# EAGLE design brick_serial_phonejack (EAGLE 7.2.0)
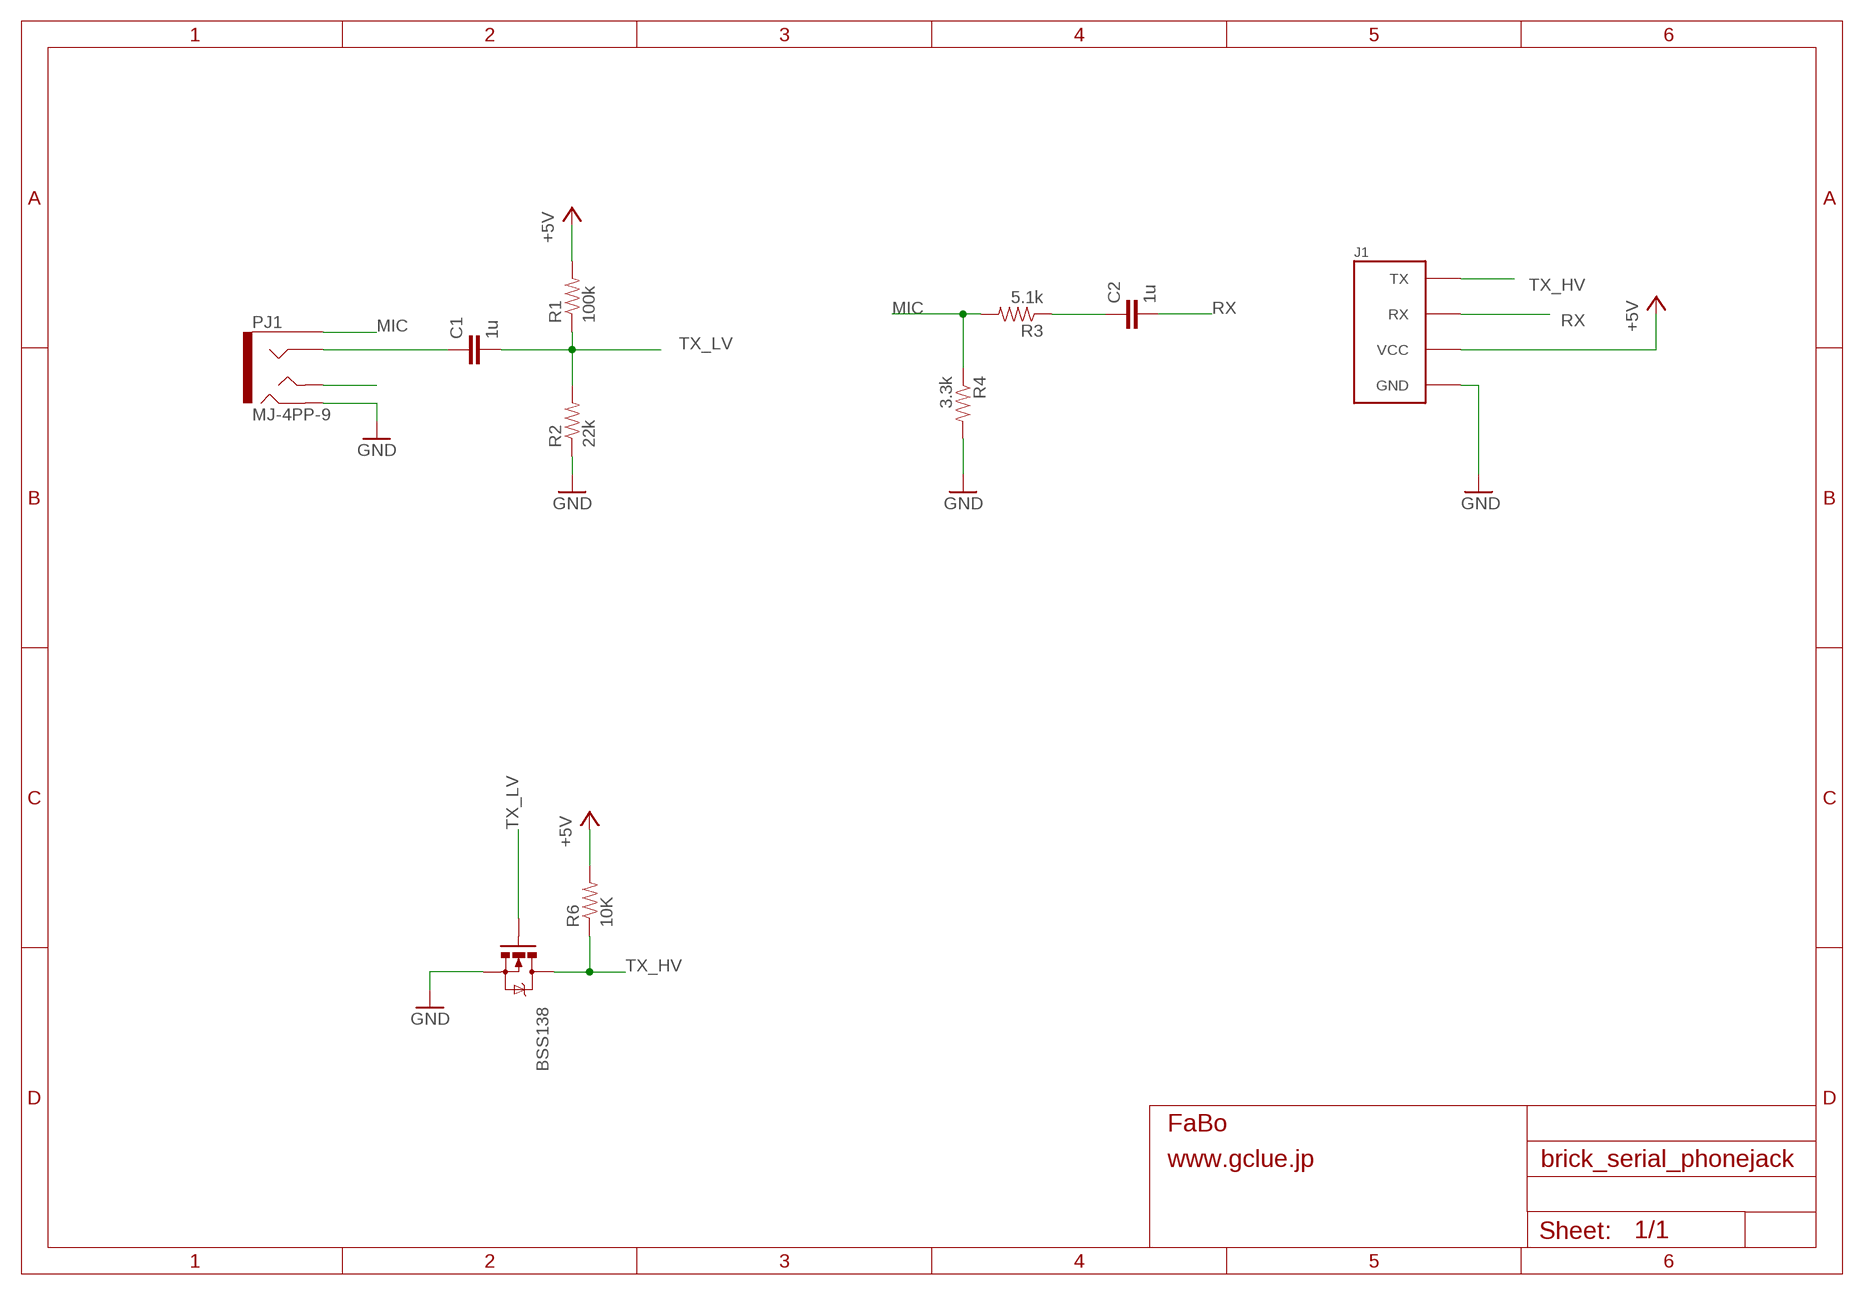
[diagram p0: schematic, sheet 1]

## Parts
BSS138  MOSFET-NCHANNELSMD  [SOT23-3]
C1  1u  CAP-EIA0603  [EIA0603-CAP]
C2  1u  CAP-EIA0603  [EIA0603-CAP]
J1  0  BRICK_SERIAL  [BRICK_SERIAL]
PJ1  MJ-4PP-9  [PHONEJACK-MJ-4PP-9]
R1  100k  RESISTOR0603  [EIA0603-RES]
R2  22k  RESISTOR0603  [EIA0603-RES]
R3  5.1k  RESISTOR0603  [EIA0603-RES]
R4  3.3k  RESISTOR0603  [EIA0603-RES]
R6  10K  RESISTOR0603-RES  [0603-RES]

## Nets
+5V: J1.VCC R1.2 R6.2
GND: BSS138.2(S) J1.GND PJ1.B R2.1 R4.2
MIC: PJ1.A R3.2 R4.1
N$1: C2.1 R3.1
N$2: C1.1 PJ1.C
N$3: PJ1.D
RX: C2.2 J1.RX
TX_HV: BSS138.3(D) J1.TX R6.1
TX_LV: BSS138.1(G) C1.2 R1.1 R2.2

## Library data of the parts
BSS138 = SparkFun:MOSFET-NCHANNEL
C1 C2 = gclue:CAP: Capacitor
J1 = gclue:BRICK_SERIAL: FaBo Brick 4pin(SERIAL)
PJ1 = gclueParts:MJ-4PP-9: 3.5mm PhoneJack 4 conductor MJ-4PP-9 http://akizukidenshi.com/download/ds/avvicon/MJ-4PP-9.pdf
R1-R4 = gclue:RESISTOR
R6 = SparkFun:RESISTOR: Resistor

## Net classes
0 default: width 0.254 mm, clearance 0.254 mm
2 gnd: width 0.305 mm, drill 0.559 mm, clearance 0.254 mm
3 usbvcc: width 0.508 mm, drill 0.61 mm, clearance 0.254 mm

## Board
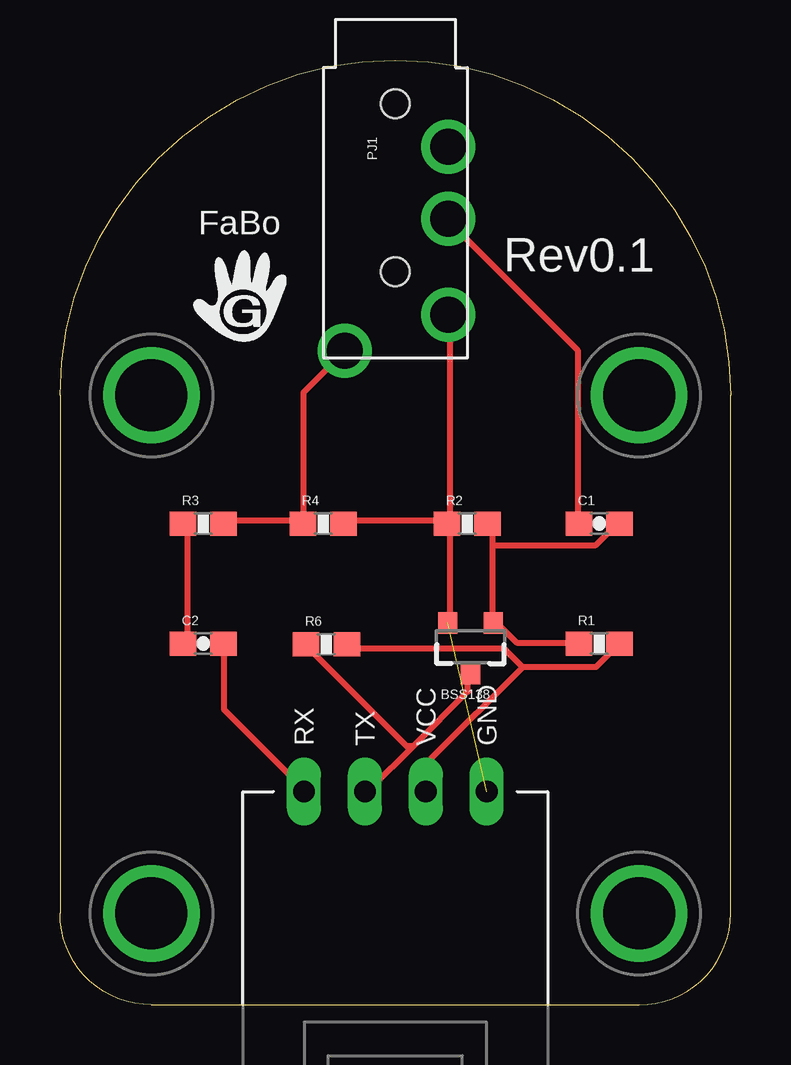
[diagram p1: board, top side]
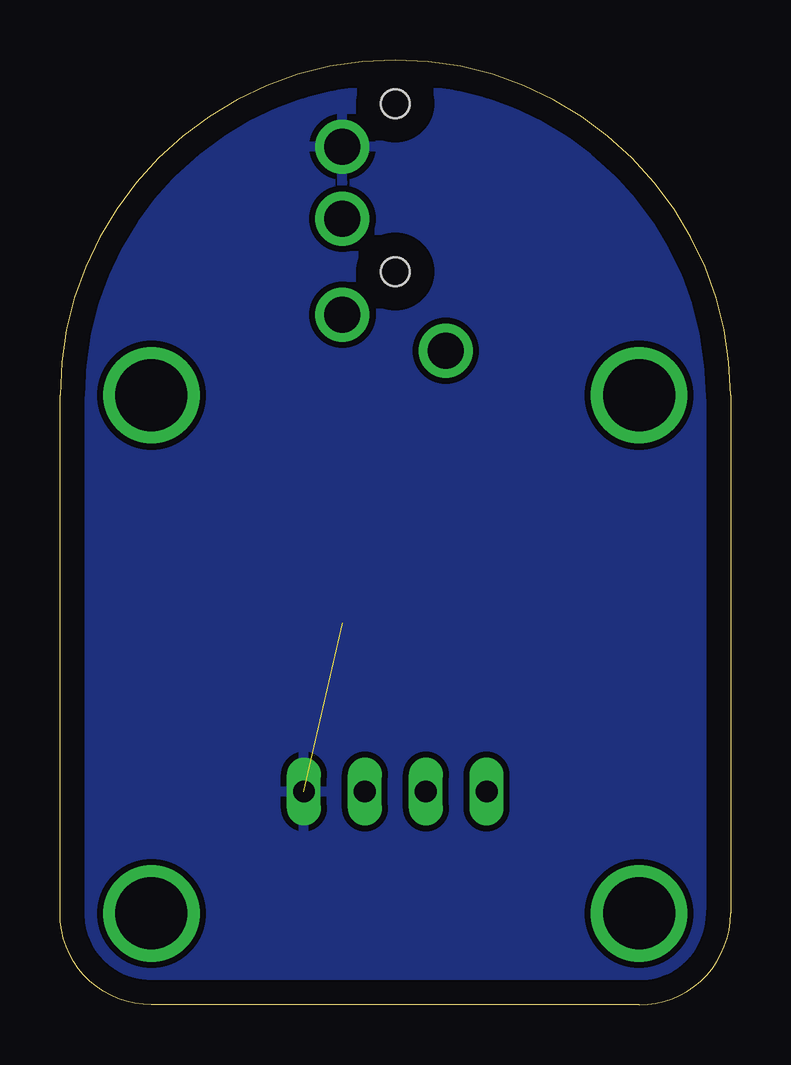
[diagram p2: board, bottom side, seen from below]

Size 27.94 x 39.37 mm. Coordinates in mm from the lower left corner, seen from the top.
Copper layers (1*16): Top 0.035mm / dielectric 1.5mm / Bottom 0.035mm
Design rules "default": minimum track width 10mil, minimum drill 24mil, track to track 8mil, track to pad 8mil, pad to pad 8mil, via to via 8mil, smd to smd 8mil, copper to edge 40mil, drill to drill 8mil, minimum pad ring 10mil, minimum via ring 8mil, stop-mask expansion 4mil, vias tented up to drill 0mil, thermal gap 10mil

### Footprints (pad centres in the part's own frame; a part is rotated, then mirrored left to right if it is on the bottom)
SOT23-3 = smd 0.8 x 0.9: 1 -0.95,-1; 2 0.95,-1; 3 0,1.1
EIA0603-CAP = smd 1.1 x 1: 1 -0.85,0; 2 0.85,0
BRICK_SERIAL = drill 0.9 long: GND 3.81,-10.16; RX -3.81,-10.16; TX -1.27,-10.16; VCC 1.27,-10.16 | drill 3 pad 3.81: P$5 -10.16,6.35; P$6 10.16,6.35; P$7 -10.16,-15.24; P$8 10.16,-15.24
PHONEJACK-MJ-4PP-9 = drill 1.5: A 5.8,-2.1; B -2.7,2.2; C 0.3,2.2; D 4.3,2.2 | hole 1.2: -4.5,0; 2.5,0
EIA0603-RES = smd 1.1 x 1: 1 -0.85,0; 2 0.85,0
0603-RES = smd 1.1 x 1: 1 -0.85,0; 2 0.85,0

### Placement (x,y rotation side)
BSS138  17.1,14.92 180 top
C1  22.47,20.05 0 top
C2  5.97,15.05 0 top
J1  13.97,19.05 0 top
PJ1  13.97,33.05 270 top
R1  22.47,15.05 0 top
R2  16.97,20.05 0 top
R3  5.97,20.05 0 top
R4  10.97,20.05 0 top
R6  11.1,15.02 0 top
U$1  [LOGO_FABO_M]  7.47,29.55 0 top

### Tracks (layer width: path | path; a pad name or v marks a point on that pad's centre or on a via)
+5V
  Top 0.254: 19.28,14.08 18.52,14.84 12.17,14.84 R6.2 | 19.28,14.08 22.33,14.08 23.09,14.84 R1.2 | 19.28,14.08 15.47,10.27 15.47,9 J1.VCC
GND  (1 unrouted)
  Top 0.254: BSS138.2 16.23,16.11 16.23,19.92 R2.1 | R4.2 11.92,20.17 15.98,20.17 R2.1 | 16.23,28.55 16.23,20.17 R2.1
  pour Bottom: -2.03,-3.95 -2.03,42.05 28.97,42.05 28.97,-3.95
MIC
  Top 0.254: R3.2 6.84,20.17 9.88,20.17 R4.1 10.14,20.17 10.14,25.51 11.66,27.03 PJ1.A
N$1
  Top 0.254: C2.1 5.31,15.09 5.31,19.92 R3.1
N$2
  Top 0.254: C1.1 21.57,20.17 21.57,27.28 16.23,32.62 PJ1.C
RX
  Top 0.254: C2.2 6.84,14.84 6.84,12.3 10.14,9 J1.RX
TX_HV
  Top 0.254: 14.71,10.77 12.93,9 J1.TX | 14.71,10.77 17,13.06 17,13.57 BSS138.3 | 14.71,10.77 14.46,10.77 10.39,14.84 R6.1
TX_LV
  Top 0.254: 18.01,19.16 18.01,19.92 R2.2 | 18.01,19.16 18.01,16.11 BSS138.1 18.27,15.85 19.03,15.09 21.57,15.09 R1.1 | 18.01,19.16 22.33,19.16 23.09,19.92 C1.2

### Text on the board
tPlace: Rev0.1

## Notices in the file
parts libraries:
SparkFun: Licensing: CC v3.0 Share-Alike You are welcome to use this library for commercial purposes.
